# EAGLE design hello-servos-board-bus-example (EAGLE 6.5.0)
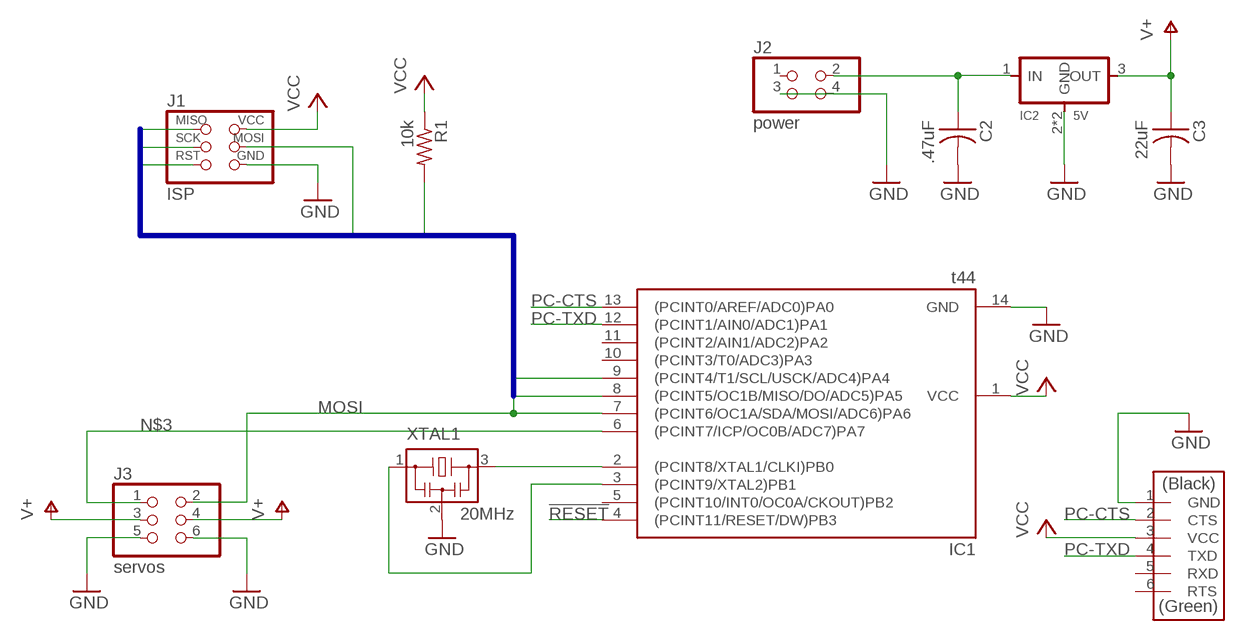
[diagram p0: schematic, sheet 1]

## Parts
C2  .47uF  CAP-US1206FAB  [C1206FAB]
C3  22uF  CAP-US1206FAB  [C1206FAB]
FTDI  FTDI-SMD-HEADER  [1X06SMD]
IC1  t44  ATTINY44-SSU  [SOIC14]
IC2  5V  REGULATORSOT223  [SOT223]
J1  ISP  AVRISPSMD  [2X03SMD]
J2  power  PINHD-2X2-SMD  [2X02SMD]
J3  servos  PINHD-2X3-SMD  [2X03SMD]
R1  10k  RES-US1206FAB  [R1206FAB]
XTAL1  20MHz  RESONATOR  [EFOBM]

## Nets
!RESET: IC1.4((PCINT11/RESET/DW)PB3) J1.5(RST) R1.2
CLK: IC1.9((PCINT4/T1/SCL/USCK/ADC4)PA4) J1.3(SCK)
GND: C2.2 C3.2 FTDI.1(GND) IC1.14(GND) IC2.2(GND) IC2.4(GND) J1.6(GND) J2.3 J2.4 J3.5 J3.6 XTAL1.2
MISO: IC1.8((PCINT5/OC1B/MISO/DO/ADC5)PA5) J1.1(MISO)
MOSI: IC1.7((PCINT6/OC1A/SDA/MOSI/ADC6)PA6) J1.4(MOSI) J3.2
N$1: IC1.2((PCINT8/XTAL1/CLKI)PB0) XTAL1.3
N$2: IC1.3((PCINT9/XTAL2)PB1) XTAL1.1
N$3: IC1.6((PCINT7/ICP/OC0B/ADC7)PA7) J3.1
N$9: C2.1 IC2.1(IN) J2.2
PC-CTS: FTDI.2(CTS) IC1.13((PCINT0/AREF/ADC0)PA0)
PC-TXD: FTDI.4(TXD) IC1.12((PCINT1/AIN0/ADC1)PA1)
V+: C3.1 IC2.3(OUT) J3.3 J3.4
VCC: FTDI.3(VCC) IC1.1(VCC) J1.2(VCC) R1.1
Unconnected: FTDI.5(RXD) FTDI.6(RTS) IC1.5((PCINT10/INT0/OC0A/CKOUT)PB2) IC1.10((PCINT3/T0/ADC3)PA3) IC1.11((PCINT2/AIN1/ADC2)PA2) J2.1

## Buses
!RESET,MISO,MOSI,CLK

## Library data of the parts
C2 C3 = fab:CAP-US
FTDI = fab:FTDI-SMD-HEADER
IC1 = fab:ATTINY44
IC2 = fab:REGULATOR
J1 = fab:AVRISP
J2 = fab:PINHD-2X2-SMD
J3 = fab:PINHD-2X3-SMD: PIN HEADER
R1 = fab:RES-US: Resistor (US Symbol)
XTAL1 = fab:RESONATOR

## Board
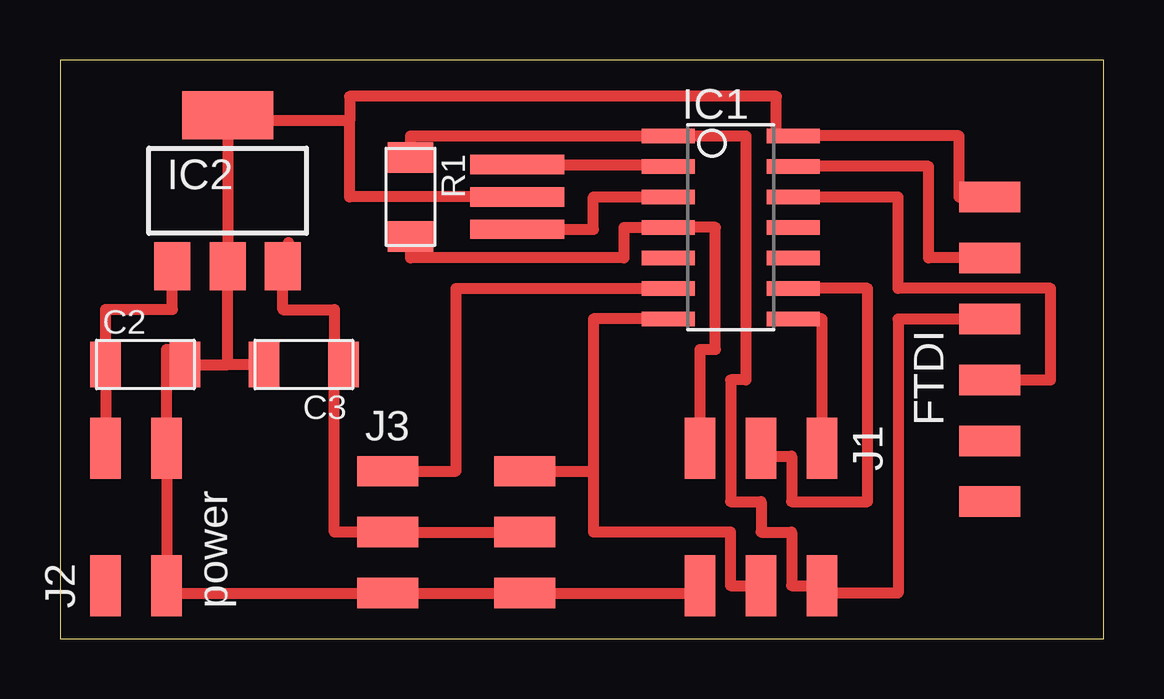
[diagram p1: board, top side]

Size 43.48 x 24.12 mm. Coordinates in mm from the lower left corner, seen from the top.
Outline: 0,0 43.48,0 43.48,24.12 0,24.12 0,0
Copper layers (1*16): Top 0.035mm / dielectric 1.5mm / Bottom 0.035mm
Design rules "design-rules-fablab": minimum track width 18mil, minimum drill 24mil, track to track 0.4mm, track to pad 0.4mm, pad to pad 0.4mm, via to via 0.4mm, smd to smd 8mil, copper to edge 1mil, drill to drill 8mil, minimum pad ring 10mil, minimum via ring 8mil, stop-mask expansion 4mil, vias tented up to drill 0mil, thermal gap 10mil

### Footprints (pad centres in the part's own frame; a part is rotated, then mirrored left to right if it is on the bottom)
C1206FAB = smd 1.27 x 1.905: 1 -1.651,0; 2 1.651,0
1X06SMD = smd 2.54 x 1.27: 1 0,6.35; 2 0,3.81; 3 0,1.27; 4 0,-1.27; 5 0,-3.81; 6 0,-6.35
SOIC14 = smd 0.61 x 2.21: 1 -3.81,-2.603; 2 -2.54,-2.603; 3 -1.27,-2.603; 4 0,-2.603; 5 1.27,-2.603; 6 2.54,-2.603; 7 3.81,-2.603; 8 3.81,2.603; 9 2.54,2.603; 10 1.27,2.603; 11 0,2.603; 12 -1.27,2.603; 13 -2.54,2.603; 14 -3.81,2.603
SOT223 = smd 1.5 x 2: 1 -2.3,-3.15; 2 0,-3.15; 3 2.3,-3.15 | smd 3.8 x 2: 4 0,3.15
2X03SMD = smd 2.54 x 1.27: 1 -2.857,2.54; 2 2.857,2.54; 3 -2.857,0; 4 2.857,0; 5 -2.857,-2.54; 6 2.857,-2.54
2X02SMD = smd 2.54 x 1.27: 1 -2.857,1.27; 2 2.857,1.27; 3 -2.857,-1.27; 4 2.857,-1.27
R1206FAB = smd 1.27 x 1.905: 1 -1.651,0; 2 1.651,0
EFOBM = smd 0.8 x 3.9: 1 -1.35,0; 2 0,0; 3 1.35,0

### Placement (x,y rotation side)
C2  3.56,11.43 0 top
C3  10.16,11.43 180 top
FTDI  38.73,12.06 0 top
IC1  27.94,17.14 270 top
IC2  6.99,18.67 0 top
J1  29.21,5.08 270 top
J2  3.17,5.08 90 top
J3  16.51,4.45 0 top
R1  14.61,18.41 270 top
XTAL1  19.05,18.41 90 top

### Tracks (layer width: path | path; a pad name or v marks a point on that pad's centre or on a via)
!RESET
  Top 0.457: R1.2 14.61,15.88 23.5,15.88 23.5,17.14 IC1.4 27.3,17.14 27.3,12.06 26.67,12.06 J1.5
CLK
  Top 0.457: J1.3 29.21,7.62 30.48,7.62 30.48,5.71 33.66,5.71 33.66,14.61 IC1.9
GND
  Top 0.457: 6.99,11.43 C2.2 5.08,11.43 5.08,12.06 4.45,12.06 J2.4 J2.3 4.45,1.91 J3.5 J3.6 26.67,1.91 J1.6 | C3.2 6.99,11.43 | 6.99,11.43 IC2.2 6.99,21.59 | XTAL1.2 12.06,18.41 12.06,21.59 | 12.06,21.59 6.99,21.59 | IC2.4 6.99,21.59 | FTDI.1 37.47,18.41 37.47,20.95 IC1.14 29.84,20.95 29.84,22.61 12.06,22.61 12.06,21.59
MISO
  Top 0.457: J1.1 31.75,13.34 IC1.8
MOSI
  Top 0.457: IC1.7 22.23,13.34 22.23,6.99 | 22.23,6.99 22.23,4.45 27.94,4.45 27.94,2.22 J1.4 | J3.2 22.23,6.99
N$1
  Top 0.457: XTAL1.3 25.34,19.77 IC1.2
N$2
  Top 0.457: XTAL1.1 22.23,17.07 22.23,18.41 IC1.3
N$3
  Top 0.457: J3.1 16.51,6.99 16.51,14.61 IC1.6
N$9
  Top 0.457: IC2.1 4.68,13.72 1.91,13.72 C2.1 J2.2
PC-CTS
  Top 0.457: FTDI.2 36.2,15.88 36.2,19.68 IC1.13
PC-TXD
  Top 0.457: FTDI.4 41.27,10.79 41.27,14.61 34.92,14.61 34.92,18.41 IC1.12
V+
  Top 0.457: J3.4 J3.3 11.43,4.45 11.43,11.43 | 9.53,16.51 9.53,15.9 IC2.3 9.29,13.72 11.43,13.72 11.43,11.43 | C3.1 11.43,11.43
VCC
  Top 0.457: FTDI.3 34.92,13.34 34.92,1.91 31.75,1.91 J1.2 30.48,2.22 30.48,4.45 29.21,4.45 29.21,5.71 27.94,5.71 27.94,10.79 28.57,10.79 28.57,20.95 IC1.1 14.61,20.95 R1.1 15.24,20.07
